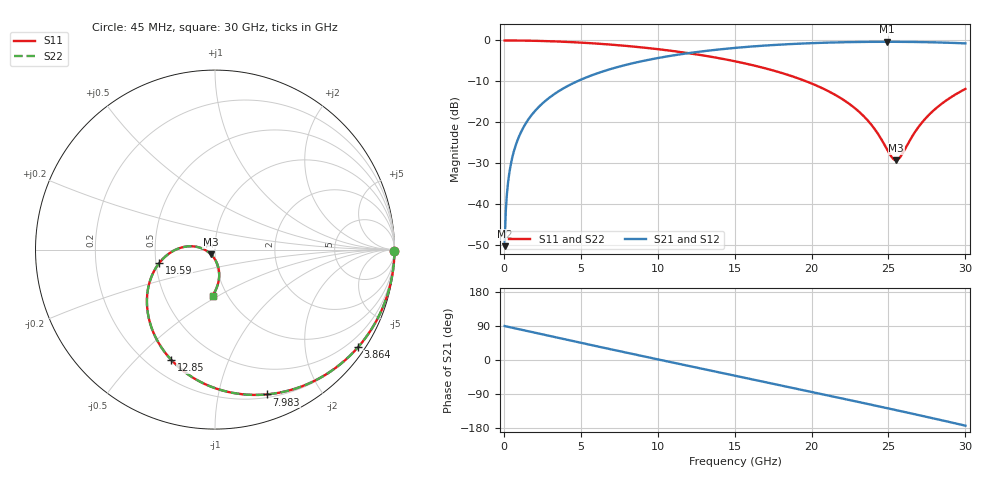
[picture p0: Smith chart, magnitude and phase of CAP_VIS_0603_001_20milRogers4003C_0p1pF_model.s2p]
! S-parameter model data by Modelithics Inc.  support@modelithics.com  813-866-6335  Tampa FL USA
! S-Parameter data specifications:
! Substrate: 20-mil Rogers 4003C, substrate thickness, H=0.508mm, Dielectric constant, Er=3.75
! PCB Mounting Pad Footprint: Pad width, PadW=0.90mm , Pad length, PadL=1.00mm , Pad gap, PadG (edge-to-edge)=1.00mm , Reference planes=3.0mm apart
! Created Wed Nov 18 13:14:53 2015
# hz S ma R 50
! 2 Port Network Data from SP1.SP block
! freq  magS11  angS11  magS21  angS21  magS12  angS12  magS22  angS22
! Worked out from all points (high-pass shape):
!   401 points, 45 MHz to 30 GHz, reference 50 ohm
!   highest |S21| = -0.33 dB at 24.91 GHz (marker M1); lowest = -50.2 dB at 45 MHz (marker M2)
!   |S21| within 3 dB of the highest: 11.57 GHz to end of sweep
!   lowest |S11| = -29.2 dB at 25.51 GHz (marker M3), VSWR 1.07, Z = 47.7 - j2.45 ohm
!   |S11| at or under -10 dB: 19.67 GHz to end of sweep
!   |S22| runs from -29.2 to 0.0 dB; largest |S21 - S12| = 0
!   S11 on the Smith chart (normalised r, x): 45 MHz: open; 3.864 GHz: 0.21, -3.22; 7.983 GHz: 0.23, -1.40; 12.85 GHz: 0.29, -0.64; 19.59 GHz: 0.52, -0.09; 30 GHz: 0.86, -0.47
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4.5e7  1 -0.4  0.003091 89.6  0.003091 89.6  1 -0.4
2.696625e8  0.9998 -2.4  0.01852 87.6  0.01852 87.6  0.9998 -2.4
4.194375e8  0.9995 -3.7  0.0288 86.2  0.0288 86.2  0.9995 -3.7
6.441e8  0.999 -5.8  0.04422 84.2  0.04422 84.2  0.999 -5.8
9.4365e8  0.9978 -8.4  0.06474 81.6  0.06474 81.6  0.9978 -8.4
2.066962e9  0.9897 -18.4  0.1411 71.5  0.1411 71.5  0.9897 -18.4
3.864262e9  0.9645 -34.4  0.2601 55.5  0.2601 55.5  0.9645 -34.4
5.062462e9  0.94 -44.9  0.3361 44.9  0.3361 44.9  0.94 -44.9
7.983075e9  0.8571 -70.3  0.5065 19.2  0.5065 19.2  0.8571 -70.3
1.007992e10  0.7802 -88.2  0.6138 1.0  0.6138 1.0  0.7802 -88.2
1.285076e10  0.6611 -111.6  0.7344 -22.9  0.7344 -22.9  0.6611 -111.6
1.50225e10  0.5571 -129.7  0.8113 -41.5  0.8113 -41.5  0.5571 -129.7
1.719424e10  0.4466 -147.5  0.8721 -60.2  0.8721 -60.2  0.4466 -147.5
1.959064e10  0.3204 -166.3  0.9207 -80.8  0.9207 -80.8  0.3204 -166.3
2.003996e10  0.2966 -169.7  0.9277 -84.7  0.9277 -84.7  0.2966 -169.7
2.303546e10  0.1376 172.2  0.9581 -110.6  0.9581 -110.6  0.1376 172.2
2.4009e10  0.0876 172.3  0.9621 -119.1  0.9621 -119.1  0.0876 172.3
2.490765e10  0.04687 -171.2  0.9633 -127.0  0.9633 -127.0  0.04687 -171.2
2.505742e10  0.0418 -164.2  0.9632 -128.4  0.9632 -128.4  0.0418 -164.2
2.550675e10  0.03466 -132.2  0.9627 -132.3  0.9627 -132.3  0.03466 -132.2
2.76036e10  0.1222 -79.5  0.9518 -151.2  0.9518 -151.2  0.1222 -79.5
3e10  0.2562 -93.0  0.9211 -173.3  0.9211 -173.3  0.2562 -93.0
